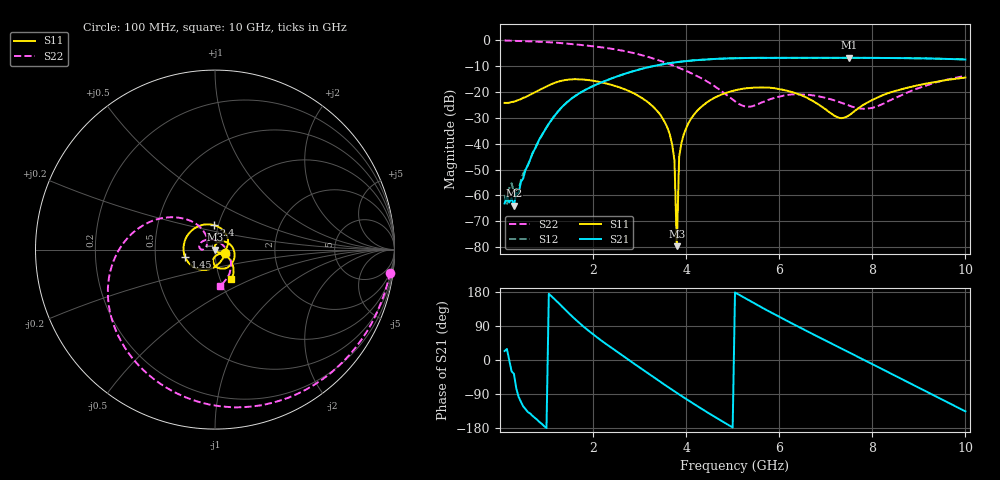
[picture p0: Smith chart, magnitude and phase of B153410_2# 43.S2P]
!  2-Port S-parameters saved by WinCal
! VAR MeasName=S-Parameters (CALIBRATED_DATA) read from VNA (N5245A)
! VAR MeasDate=2016-12-23 10:01:35
! VAR NAME=B153410_2# 43
! VAR FILENAME=B153410_2# 43.S2P
! VAR DATE=2016-12-23 10:01:35
! VAR PHYS_PORTS=1,2
# Hz S DB R 50
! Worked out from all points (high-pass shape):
!   199 points, 100 MHz to 10 GHz, reference 50 ohm
!   highest |S21| = -6.83 dB at 7.5 GHz (marker M1); lowest = -64.0 dB at 300 MHz (marker M2)
!   |S21| within 3 dB of the highest: 3.352 GHz to end of sweep
!   lowest |S11| = -79.6 dB at 3.8 GHz (marker M3), VSWR 1.00, Z = 50 + j0.00618 ohm
!   |S11| at or under -10 dB: start of sweep to end of sweep
!   |S22| runs from -26.5 to -0.1 dB; largest |S21 - S12| = 0.0025
!   S11 on the Smith chart (normalised r, x): 100 MHz: 1.12, -0.05; 1.45 GHz: 0.71, -0.06; 2.4 GHz: 0.95, +0.26; 10 GHz: 1.12, -0.39
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1e8  -24.24 -19.2  -63.08 23.7  -59.77 16.2  -0.13 -7.5
1.5e8  -24.26 -26.0  -60.36 28.9  -63.55 33.9  -0.18 -10.9
2.5e8  -23.89 -40.0  -61.03 -30.1  -55.30 -25.0  -0.25 -17.6
3e8  -23.78 -46.6  -63.99 -36.3  -58.77 -44.2  -0.28 -21.0
8.5e8  -19.24 -102.6  -38.18 -163.6  -38.43 -164.5  -0.63 -57.1
1.45e9  -15.29 -167.0  -23.86 127.1  -23.88 127.1  -1.35 -95.0
1.75e9  -15.16 159.8  -20.05 92.9  -20.06 93.0  -1.88 -112.8
2.4e9  -17.28 92.6  -14.78 31.7  -14.78 31.7  -3.34 -149.4
3.4e9  -27.81 -19.4  -9.66 -53.7  -9.64 -53.7  -7.72 159.5
3.65e9  -36.49 -47.9  -8.89 -74.6  -8.87 -74.5  -9.31 149.1
3.75e9  -46.58 -65.5  -8.63 -82.7  -8.62 -82.7  -10.01 145.4
3.8e9  -79.58 143.9  -8.51 -86.8  -8.50 -86.7  -10.37 143.4
3.85e9  -45.08 111.7  -8.40 -90.9  -8.39 -90.8  -10.72 141.7
3.95e9  -36.33 98.4  -8.20 -98.9  -8.18 -98.8  -11.48 138.4
4.35e9  -25.39 56.9  -7.55 -130.0  -7.55 -130.1  -14.94 126.5
5.05e9  -19.38 -5.4  -6.98 178.3  -6.99 178.4  -23.66 131.6
5.95e9  -18.77 -67.3  -6.86 117.4  -6.84 117.5  -22.01 178.3
6.7e9  -23.26 -98.2  -6.84 69.8  -6.84 69.8  -21.27 152.3
7.5e9  -29.07 -44.2  -6.83 20.1  -6.84 20.1  -25.24 97.5
8.35e9  -20.40 -32.4  -6.91 -32.7  -6.90 -32.5  -23.50 -2.2
9.15e9  -16.84 -44.9  -7.06 -82.4  -7.07 -82.4  -17.56 -48.6
1e10  -14.47 -61.9  -7.49 -135.6  -7.48 -135.3  -13.87 -82.5
